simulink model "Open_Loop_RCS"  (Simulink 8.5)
settings: Solver=ode4  StartTime=0.0  StopTime=3000  FixedStep=Ts  RelTol=1e-3
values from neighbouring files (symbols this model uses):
  Ave = [    [vehicle_flex34.m]    (also in vehicle_rigid.m)
  Bve = [    [vehicle_flex34.m]    (also in vehicle_rigid.m)
  CB2L = [cpsi, -cphi*spsi,  sphi*spsi;          0,    cphi,      -sphi;          0,    sphi*cpsi,  cphi*cpsi]/cpsi    [Rigbod_Dynam_LVLH.m]    (also in start.m = eye(3); start2.m = eye(3); start3.m = eye(3); start1.m = eye(3))
  Cve = [    [vehicle_flex34.m]    (also in vehicle_rigid.m)
  Dve = [    [vehicle_flex34.m]    (also in vehicle_rigid.m)
  ini = [wbo; atto; Hco]    [start.m]    (also in start2.m; start3.m; start1.m)
  Na_max = 0.636/(deadband(1)*d2r)    [start.m]    (also in start2.m; start3.m; Dead_Band_DF.m = 72.8802315406)
  nt = 12    [start.m]    (also in start2.m; start3.m; start1.m)
  wo = 0.0011    [start.m]    (also in start2.m; start3.m; start1.m)
undefined symbols (not defined in the file or in its folder): JSel_ln, Mix, Rigbod_Dynam_LVLH, UnitV

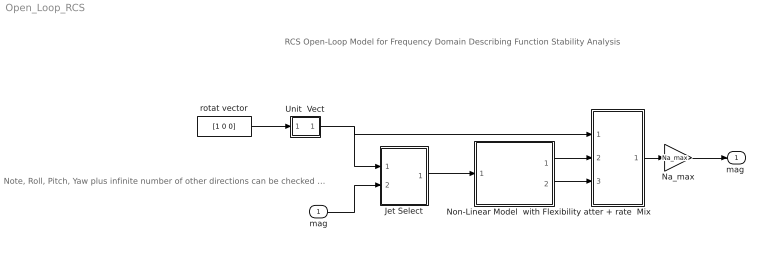
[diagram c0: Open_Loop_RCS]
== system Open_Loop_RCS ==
  note: RCS Open-Loop Model for Frequency Domain Describing Function Stability Analysis
  note: Note, Roll, Pitch, Yaw plus infinite number of other directions can be checked for Stability Each direction corresponds to a unique set of thrusters
  mag : Inport  PortDimensions=1
  Jet Select : Subsystem
  Na_max : Gain  Gain=Na_max
  Non-Linear Model  with Flexibility : Subsystem
  Unit  Vect : Subsystem
  atter + rate  Mix : Subsystem
  rotat vector : Constant  Value=[1 0 0]
  "mag " : Outport
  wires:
  Non-Linear Model  with Flexibility/1(atti) -> atter + rate  Mix/2(atter)
  Non-Linear Model  with Flexibility/2(w-lv) -> atter + rate  Mix/3(rater)
  mag/1 -> Jet Select/2(mag)
  Unit  Vect/1(U) -> Jet Select/1(Udir), atter + rate  Mix/1(Udir)
  rotat vector/1 -> Unit  Vect/1(V)
  atter + rate  Mix/1(mag) -> Na_max/1
  Na_max/1 -> "mag "/1
  Jet Select/1(f(i)) -> Non-Linear Model  with Flexibility/1(Frcs)

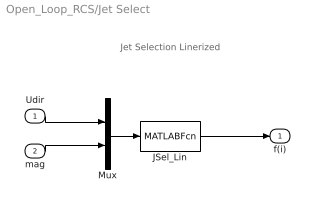
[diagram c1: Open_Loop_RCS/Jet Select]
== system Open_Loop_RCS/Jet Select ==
  note: Jet Selection Linerized
  Udir : Inport
  mag : Inport  Port=2
  JSel_Lin : MATLABFcn  MATLABFcn=JSel_ln( u(1:3), u(4) )  OutputDimensions=nt
  Mux : Mux  Inputs="[3  1]"
  f(i) : Outport
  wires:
  Mux/1 -> JSel_Lin/1
  JSel_Lin/1 -> f(i)/1
  Udir/1 -> Mux/1
  mag/1 -> Mux/2

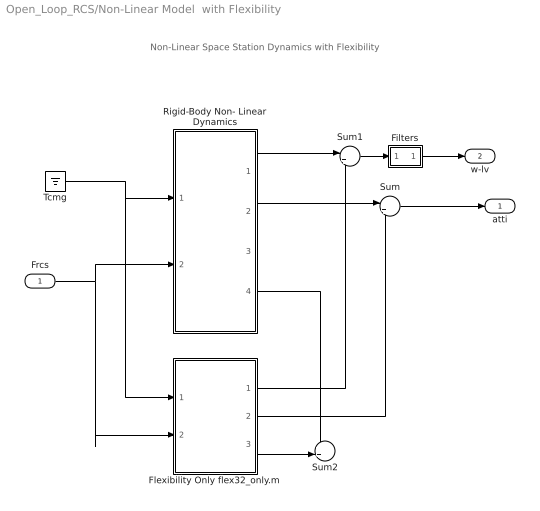
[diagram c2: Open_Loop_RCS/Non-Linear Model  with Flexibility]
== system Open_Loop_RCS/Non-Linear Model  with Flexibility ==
  note: Non-Linear Space Station Dynamics with Flexibility
  Frcs : Inport
  Filters : Subsystem
  Flexibility Only flex32_only.m : Subsystem
  Rigid-Body Non- Linear Dynamics : Subsystem
  Sum : Sum  Inputs=|++
  Sum1 : Sum  Inputs=|++
  Sum2 : Sum  Inputs=++|
  Tcmg : Ground
  atti : Outport
  w-lv : Outport  Port=2
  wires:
  Frcs/1 -> Rigid-Body Non- Linear Dynamics/2(Frcs), Flexibility Only flex32_only.m/2(Frcs)
  Rigid-Body Non- Linear Dynamics/2(atti-lv) -> Sum/1
  Flexibility Only flex32_only.m/2(att) -> Sum/2
  Sum/1 -> atti/1
  Sum1/1 -> Filters/1(I)
  Tcmg/1 -> Rigid-Body Non- Linear Dynamics/1(Tcmg), Flexibility Only flex32_only.m/1(Tcmg)
  Rigid-Body Non- Linear Dynamics/1(w-lv) -> Sum1/1
  Flexibility Only flex32_only.m/1(wbf) -> Sum1/2
  Flexibility Only flex32_only.m/3(wb) -> Sum2/2
  Rigid-Body Non- Linear Dynamics/4(wb) -> Sum2/1
  Filters/1(O) -> w-lv/1

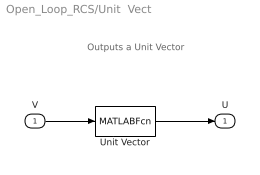
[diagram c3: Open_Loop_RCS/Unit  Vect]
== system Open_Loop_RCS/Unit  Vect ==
  note: Outputs a Unit Vector
  V : Inport
  Unit Vector : MATLABFcn  MATLABFcn=UnitV( u(1:3) )  OutputDimensions=3
  U : Outport
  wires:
  Unit Vector/1 -> U/1
  V/1 -> Unit Vector/1

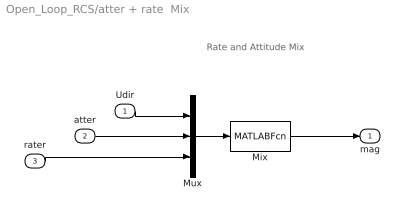
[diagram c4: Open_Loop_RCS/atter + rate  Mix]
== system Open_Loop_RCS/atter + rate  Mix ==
  note: Rate and Attitude Mix
  Udir : Inport
  atter : Inport  Port=2
  rater : Inport  Port=3
  Mix : MATLABFcn  MATLABFcn=Mix( u(1:3), u(4:6), u(7:9) )  OutputDimensions=1
  Mux : Mux  Inputs="[3  3  3]"
  mag : Outport
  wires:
  rater/1 -> Mux/3
  Mux/1 -> Mix/1
  Udir/1 -> Mux/1
  atter/1 -> Mux/2
  Mix/1 -> mag/1

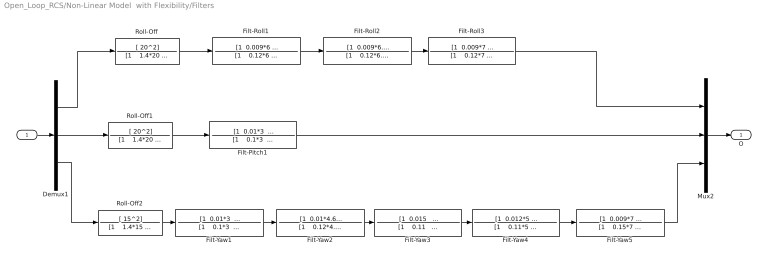
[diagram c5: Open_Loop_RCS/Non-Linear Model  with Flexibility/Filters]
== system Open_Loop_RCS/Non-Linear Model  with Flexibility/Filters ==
  I : Inport
  Demux1 : Demux  Outputs=3
  Filt-Pitch1 : TransferFcn  Numerator="[1  0.01*3   3.07^2]"  Denominator="[1    0.1*3    3.07^2]"
  Filt-Roll1 : TransferFcn  Numerator="[1  0.009*6   5.85^2]"  Denominator="[1    0.12*6    5.85^2]"
  Filt-Roll2 : TransferFcn  Numerator="[1  0.009*6.4   6.46^2]"  Denominator="[1    0.12*6.4    6.46^2]"
  Filt-Roll3 : TransferFcn  Numerator="[1  0.009*7   7.51^2]"  Denominator="[1    0.12*7    7.51^2]"
  Filt-Yaw1 : TransferFcn  Numerator="[1  0.01*3   3.07^2]"  Denominator="[1    0.1*3    3.07^2]"
  Filt-Yaw2 : TransferFcn  Numerator="[1  0.01*4.6   4.6^2]"  Denominator="[1    0.12*4.6    4.6^2]"
  Filt-Yaw3 : TransferFcn  Numerator="[1  0.015   1.14^2]"  Denominator="[1    0.11    1.14^2]"
  Filt-Yaw4 : TransferFcn  Numerator="[1  0.012*5   5.21^2]"  Denominator="[1    0.11*5    5.21^2]"
  Filt-Yaw5 : TransferFcn  Numerator="[1  0.009*7   6.83^2]"  Denominator="[1    0.15*7    6.83^2]"
  Mux2 : Mux  Inputs=3
  Roll-Off : TransferFcn  Numerator=[ 20^2]  Denominator="[1    1.4*20    20^2]"
  Roll-Off1 : TransferFcn  Numerator=[ 20^2]  Denominator="[1    1.4*20    20^2]"
  Roll-Off2 : TransferFcn  Numerator=[ 15^2]  Denominator="[1    1.4*15    15^2]"
  O : Outport
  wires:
  I/1 -> Demux1/1
  Mux2/1 -> O/1
  Demux1/1 -> Roll-Off/1
  Demux1/3 -> Roll-Off2/1
  Demux1/2 -> Roll-Off1/1
  Roll-Off/1 -> Filt-Roll1/1
  Roll-Off2/1 -> Filt-Yaw1/1
  Roll-Off1/1 -> Filt-Pitch1/1
  Filt-Roll1/1 -> Filt-Roll2/1
  Filt-Roll2/1 -> Filt-Roll3/1
  Filt-Roll3/1 -> Mux2/1
  Filt-Pitch1/1 -> Mux2/2
  Filt-Yaw1/1 -> Filt-Yaw2/1
  Filt-Yaw2/1 -> Filt-Yaw3/1
  Filt-Yaw3/1 -> Filt-Yaw4/1
  Filt-Yaw4/1 -> Filt-Yaw5/1
  Filt-Yaw5/1 -> Mux2/3

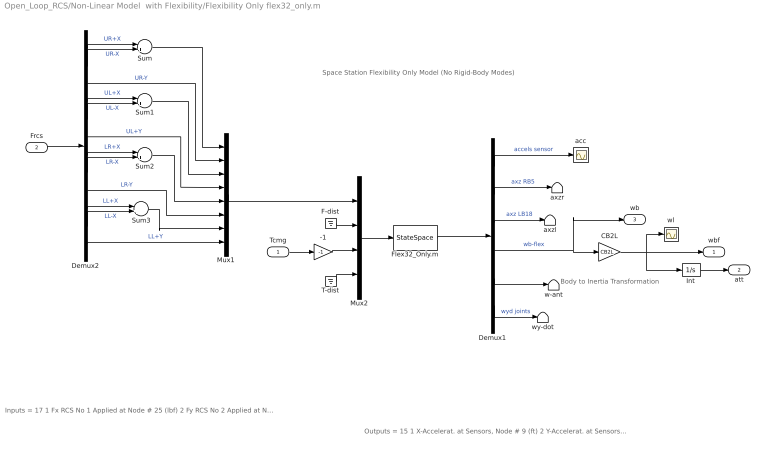
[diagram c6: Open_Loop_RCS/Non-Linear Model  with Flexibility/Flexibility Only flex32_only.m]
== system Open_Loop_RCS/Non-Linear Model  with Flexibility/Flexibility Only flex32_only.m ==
  note: Outputs = 15 1 X-Accelerat. at Sensors, Node # 9 (ft) 2 Y-Accelerat. at Sensors, Node # 9 (ft) 3 Z-Accelerat. at Sensors, Node # 9 (ft) 4 X-Accelerat. at Right Boom End, Node # 5 (ft) 5 Z-Accelerat. at Right Boom End, Node # 5 (ft) 6 X-Accelerat. at Left Boom End, Node # 18 (ft) 7 Z-Accelerat. at Left Boom End, Node # 18 (ft) 8 X-Rot. Rate at Sensors, Node # 9 (radian) 9 Y-Rot. Rate at Sensors, Node # 9 (radian) 10 Z-Rot. Rate at Sensors, Node # 9 (radian) 11 X-Rot. Rate at Antena Bot-Left, Node # 24 (radian) 12 Y-Rot. Rate at Antena Bot-Left, Node # 24 (radian) 13 Z-Rot. Rate at Antena Bot-Left, Node # 24 (radian) 14 Y-Rot.Accel. at Right Joint, Node # 7 (radian) 15 Y-Rot.Accel. at Left Joint, Node # 16 (radian)
  note: Inputs = 17 1 Fx RCS No 1 Applied at Node # 25 (lbf) 2 Fy RCS No 2 Applied at Node # 25 (lbf) 3 Fx RCS No 3 Applied at Node # 26 (lbf) 4 Fy RCS No 4 Applied at Node # 26 (lbf) 5 Fx RCS No 5 Applied at Node # 27 (lbf) 6 Fy RCS No 6 Applied at Node # 27 (lbf) 7 Fx RCS No 7 Applied at Node # 28 (lbf) 8 Fy RCS No 8 Applied at Node # 28 (lbf) 9 Fx Disturb. No 9 at Node # 21 (lbf) 10 Fy Disturb. No 10 at Node # 21 (lbf) 11 Fz Disturb. No 11 at Node # 21 (lbf) 12 Torq-x No 1 CMG Applied at Node # 10 (ft-lb) 13 Torq-y No 2 CMG Applied at Node # 10 (ft-lb) 14 Torq-z No 3 CMG Applied at Node # 10 (ft-lb) 15 Torq-x No 4 Gimbal Dist. at Node # 1 (ft-lb) 16 Torq-y No 5 Gimbal Dist. at Node # 1 (ft-lb) 17 Torq-z No 6 Gimbal Dist. at Node # 1 (ft-lb)
  note: Space Station Flexibility Only Model (No Rigid-Body Modes)
  note: Body to Inertia Transformation
  Tcmg : Inport
  Frcs : Inport  Port=2
  -1 : Gain  Gain=-1
  CB2L : Gain  Gain=CB2L  Multiplication=Matrix(K*u)
  Demux1 : Demux  Outputs=[3, 2, 2, 3, 3, 2]
  Demux2 : Demux  Outputs=12
  F-dist : Ground
  Flex32_Only.m : StateSpace  A=Ave  B=Bve  C=Cve  D=Dve  X0=0
  Int : Integrator
  Mux1 : Mux  Inputs=8
  Mux2 : Mux  Inputs=[8, 3, 3, 3]
  Sum{,1..3} (4 alike) : Sum  Inputs=|+-
  T-dist : Ground
  acc : Scope
  axzl : Terminator
  axzr : Terminator
  w-ant : Terminator
  wl : Scope
  wy-dot : Terminator
  wbf : Outport
  att : Outport  Port=2
  wb : Outport  Port=3
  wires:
  Demux1/6 -> wy-dot/1  "wyd joints"
  Demux1/5 -> w-ant/1
  T-dist/1 -> Mux2/4
  F-dist/1 -> Mux2/2
  Demux1/3 -> axzl/1  "axz LB18"
  Demux1/2 -> axzr/1  "axz RB5"
  Tcmg/1 -> -1/1
  Demux1/4 -> CB2L/1, wb/1  "wb-flex"
  Demux1/1 -> acc/1  "accels sensor"
  Flex32_Only.m/1 -> Demux1/1
  Mux2/1 -> Flex32_Only.m/1
  Mux1/1 -> Mux2/1
  Frcs/1 -> Demux2/1
  Demux2/6 -> Mux1/4  "UL+Y"
  Demux2/9 -> Mux1/6  "LR-Y"
  Demux2/12 -> Mux1/8  "LL+Y"
  Demux2/3 -> Mux1/2  "UR-Y"
  Demux2/1 -> Sum/1  "UR+X"
  Demux2/2 -> Sum/2  "UR-X"
  Sum/1 -> Mux1/1
  Demux2/4 -> Sum1/1  "UL+X"
  Demux2/5 -> Sum1/2  "UL-X"
  Sum1/1 -> Mux1/3
  Demux2/7 -> Sum2/1  "LR+X"
  Demux2/8 -> Sum2/2  "LR-X"
  Demux2/10 -> Sum3/1  "LL+X"
  Demux2/11 -> Sum3/2  "LL-X"
  Sum3/1 -> Mux1/7
  Sum2/1 -> Mux1/5
  Int/1 -> att/1
  -1/1 -> Mux2/3
  CB2L/1 -> wl/1, wbf/1, Int/1

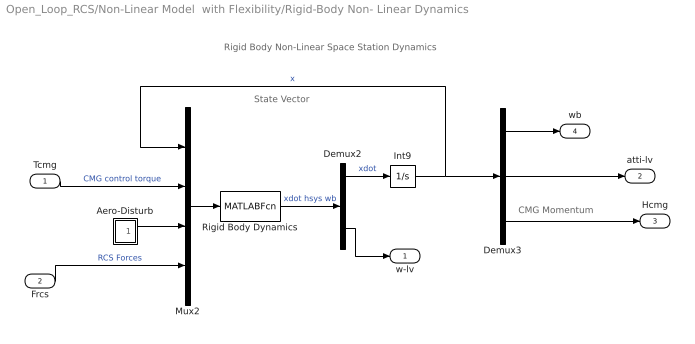
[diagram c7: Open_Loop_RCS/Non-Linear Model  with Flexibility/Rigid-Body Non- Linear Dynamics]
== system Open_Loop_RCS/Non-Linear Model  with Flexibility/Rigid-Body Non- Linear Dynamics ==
  note: CMG Momentum
  note: State Vector
  note: Rigid Body Non-Linear Space Station Dynamics
  Tcmg : Inport  PortDimensions=3
  Frcs : Inport  Port=2  PortDimensions=nt
  Aero-Disturb : Subsystem
  Demux2 : Demux  Outputs=[9,3,3]
  Demux3 : Demux  Outputs=[3,3,3]
  Int9 : Integrator  InitialCondition=ini
  Mux2 : Mux  Inputs=[9, 3, 3, nt]
  Rigid Body Dynamics : MATLABFcn  MATLABFcn=Rigbod_Dynam_LVLH( u(1:9), u(10:12), u(13:15), u(16:15+nt) )  OutputDimensions=15
  w-lv : Outport
  atti-lv : Outport  Port=2
  Hcmg : Outport  Port=3
  wb : Outport  Port=4
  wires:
  Mux2/1 -> Rigid Body Dynamics/1
  Frcs/1 -> Mux2/4  "RCS Forces"
  Demux3/3 -> Hcmg/1
  Demux3/2 -> atti-lv/1
  Demux2/3 -> w-lv/1
  Tcmg/1 -> Mux2/2  "CMG control torque"
  Int9/1 -> Mux2/1, Demux3/1  "x"
  Demux2/1 -> Int9/1  "xdot"
  Rigid Body Dynamics/1 -> Demux2/1  "xdot hsys wb"
  Aero-Disturb/1(Td) -> Mux2/3
  Demux3/1 -> wb/1

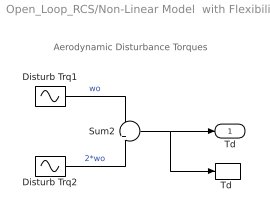
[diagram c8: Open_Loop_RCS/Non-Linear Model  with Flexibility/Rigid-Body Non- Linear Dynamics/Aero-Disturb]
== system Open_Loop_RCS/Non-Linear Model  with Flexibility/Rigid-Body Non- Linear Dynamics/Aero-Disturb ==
  note: Aerodynamic Disturbance Torques
  Disturb Trq1 : Sin  Amplitude=[1, 3, 1]  Bias="[1  8  1]"  Frequency=[wo, wo, wo]  SampleTime=0
  Disturb Trq2 : Sin  Amplitude=[1, 1, 1]*0.5  Frequency=[wo, wo, wo]*2  SampleTime=0
  Sum2 : Sum  Inputs=+|+
  "Td " : ToWorkspace  VariableName=Td  SampleTime=-1
  Td : Outport
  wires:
  Disturb Trq2/1 -> Sum2/2  "2*wo"
  Sum2/1 -> "Td "/1, Td/1
  Disturb Trq1/1 -> Sum2/1  "wo"
